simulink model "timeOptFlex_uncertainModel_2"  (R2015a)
settings: Solver=ode3  StartTime=0.0  StopTime=trun  FixedStep=step_sz  RelTol=1e-3
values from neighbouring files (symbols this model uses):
  bobar = 1.01*bo    (= 18458760)    [results.m]
  c = bo/w^2    (= 4.59233914625)    [figure_4.m]    (also in figure_3.m; figure_2.m; results.m)
  step_sz = .00000006    (= 6e-08)    [figure_4.m]    (also in figure_2.m = 6e-07; results.m = 1e-07)
  w = 2*pi*3.175*10^2    (= 1994.91133503)    [figure_4.m]    (also in figure_3.m; figure_2.m; results.m; plotshaded.m = varargout)
  wbar = 0.99*w    (= 1974.96222168)    [results.m]
  x1Tol = .001*c    (= 0.00459233914625)    [figure_4.m]    (also in figure_2.m = 2.6e-12; results.m)
  x2Tol = .00001    (= 1e-05)    [figure_2.m]    (also in results.m = 9.16130941716)
  Xo = [8.665 4229]    [figure_4.m]    (also in figure_3.m = [2*c, 0]; figure_2.m = [curves_optx1(k), curves_optx2(k)]; results.m = [3.0*c,0])
libraries: simulink x2, commnoisgen2 x1

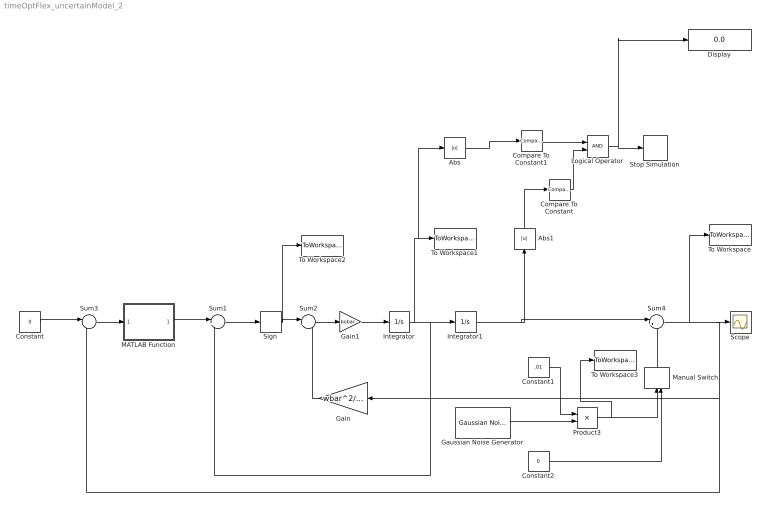
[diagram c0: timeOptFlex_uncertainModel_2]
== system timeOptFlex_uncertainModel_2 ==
  Abs : Abs
  Abs1 : Abs
  Compare To Constant : simulink/Logic and Bit Operations/Compare To Constant  relop=<  const=x1Tol  OutDataTypeStr=boolean
  Compare To Constant1 : simulink/Logic and Bit Operations/Compare To Constant  relop=<  const=x2Tol  OutDataTypeStr=boolean
  Constant : Constant  Value=0
  Constant1 : Constant  Value=.01
  Constant2 : Constant  Value=0
  Display : Display
  Gain : Gain  Gain=wbar^2/bobar
  Gain1 : Gain  Gain=bobar
  Gaussian Noise Generator : commnoisgen2/Gaussian Noise Generator  m=0  d=1  s=41  Ts=step_sz  frameBased=off  sampPerFrame=1  orient=off  outDataType=double
  Integrator : Integrator  InitialCondition=Xo(2)
  Integrator1 : Integrator  InitialCondition=Xo(1)
  Logical Operator : Logic  AllPortsSameDT=off  OutDataTypeStr=boolean
  MATLAB Function : MATLAB Function  TreatAsAtomicUnit=on
  Manual Switch : ManualSwitch  CurrentSetting=0
  Product3 : Product
  Scope : Scope
  Sign : Signum
  Stop Simulation : Stop
  Sum1 : Sum  Inputs=|+-
  Sum2 : Sum  Inputs=|+-
  Sum3 : Sum  Inputs=|+-
  Sum4 : Sum  Inputs=|++
  To Workspace : ToWorkspace  VariableName=x1_uncertain  SampleTime=-1
  To Workspace1 : ToWorkspace  VariableName=x2_uncertain  SampleTime=-1
  To Workspace2 : ToWorkspace  VariableName=u_opt  SampleTime=-1
  To Workspace3 : ToWorkspace  VariableName=gauss_out  SampleTime=-1
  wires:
  Gain/1 -> Sum2/2
  Gain1/1 -> Integrator/1
  Sum1/1 -> Sign/1
  Sum2/1 -> Gain1/1
  Sign/1 -> To Workspace2/1, Sum2/1
  MATLAB Function/1(y) -> Sum1/1
  Sum3/1 -> MATLAB Function/1(u)
  Constant/1 -> Sum3/1
  Integrator1/1 -> Abs1/1, Sum4/1
  Sum4/1 -> To Workspace/1, Gain/1, Sum3/2, Scope/1
  Gaussian Noise Generator/1 -> Product3/2
  Constant1/1 -> Product3/1
  Manual Switch/1 -> Sum4/2
  Product3/1 -> To Workspace3/1, Manual Switch/1
  Constant2/1 -> Manual Switch/2
  Integrator/1 -> Abs/1, To Workspace1/1, Sum1/2, Integrator1/1
  Compare To Constant1/1 -> Logical Operator/1
  Compare To Constant/1 -> Logical Operator/2
  Logical Operator/1 -> Display/1, Stop Simulation/1
  Abs/1 -> Compare To Constant1/1
  Abs1/1 -> Compare To Constant/1

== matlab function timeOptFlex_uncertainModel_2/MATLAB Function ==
function y = fcn(u, c, w)
%#codegen


if (mod(sign(u(1)/c)*floor(abs(u(1)/c)), 2)==0);
% if (mod(sign(u(1)/c)*floor(abs(u(1)/c)), 2)==0);    
%         x1_bar=c-abs(fpart*c);
       x1_bar=c-abs(fracpart(u(1)/c)*c);
%        x1_bar=c-abs(fracpart(u(1)/c)*c);
    else
%         x1_bar=fpart*c;
        x1_bar=fracpart(u(1)/c)*c;
%         x1_bar=fracpart(u(1)/c)*c;
end


% x2_opt(i)=-sign(x1_opt(i))*(bo/w)*sqrt(1-(w^4)*(x1_bar(i))^2/(bo^2));

fx=sign(u(1))*w*sqrt(c^2 -x1_bar^2 );






y = fx;
